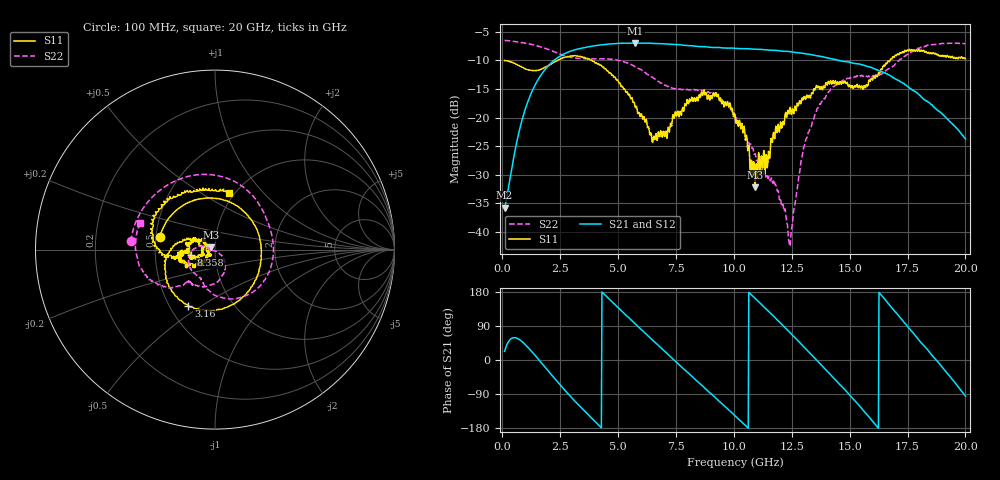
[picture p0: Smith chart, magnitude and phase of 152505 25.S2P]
!  2-Port S-parameters saved by WinCal
! VAR MeasName=S-Parameters (CALIBRATED_DATA) read from VNA (N5230C)
! VAR MeasDate=4/10/2015 9:30:51 AM
! VAR NAME=152505 25
! VAR FILENAME=152505 25.S2P
! VAR DATE=4/10/2015 9:30:51 AM
! VAR PHYS_PORTS=1,2
# Hz S DB R 50
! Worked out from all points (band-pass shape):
!   801 points, 100 MHz to 20 GHz, reference 50 ohm
!   highest |S21| = -6.97 dB at 5.747 GHz (marker M1); lowest = -35.7 dB at 100 MHz (marker M2)
!   |S21| within 3 dB of the highest: 2.252 GHz to 14.49 GHz (12.24 GHz wide, 146 % of centre)
!   lowest |S11| = -32.2 dB at 10.92 GHz (marker M3), VSWR 1.05, Z = 48 + j1.26 ohm
!   |S11| at or under -10 dB: start of sweep to 2.393 GHz; 3.863 GHz to 16.74 GHz (12.88 GHz wide, 125 % of centre)
!   |S22| runs from -42.5 to -6.5 dB; largest |S21 - S12| = 0.0073
!   S11 on the Smith chart (normalised r, x): 100 MHz: 0.53, +0.08; 3.16 GHz: 0.62, -0.44; 8.358 GHz: 0.76, -0.05; 20 GHz: 0.94, +0.67
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1e8  -10.05 166.8  -35.72 22.8  -35.60 22.2  -6.55 174.3
6.72125e8  -10.86 91.6  -23.40 56.3  -23.39 56.2  -6.80 142.2
1.44325e9  -11.79 5.7  -14.11 10.2  -14.11 10.2  -7.41 100.9
2.214375e9  -10.36 -55.5  -10.09 -45.4  -10.09 -45.4  -8.48 62.4
3.159625e9  -9.17 -115.3  -8.15 -110.2  -8.14 -110.3  -9.62 24.4
3.43325e9  -9.40 -130.4  -7.89 -127.5  -7.88 -127.5  -9.72 14.2
4.52775e9  -11.86 -176.8  -7.20 166.2  -7.21 166.0  -9.78 -28.9
5.746625e9  -18.29 156.5  -6.97 94.9  -7.03 94.9  -11.17 -78.3
6.741625e9  -22.49 -179.1  -7.08 38.2  -7.08 38.0  -13.73 -107.6
8.3585e9  -17.18 -167.8  -7.55 -52.9  -7.54 -52.5  -15.21 -135.3
9.179375e9  -16.28 166.8  -7.76 -98.0  -7.73 -98.0  -16.00 -159.6
1.005e10  -19.53 151.0  -7.91 -147.3  -7.93 -147.3  -19.82 172.8
1.092062e10  -32.20 147.5  -8.07 162.5  -8.07 162.8  -26.29 163.7
1.181612e10  -21.51 -131.8  -8.28 109.4  -8.28 108.9  -31.81 -167.5
1.2438e10  -18.22 -132.3  -8.52 71.3  -8.57 71.0  -42.37 -86.5
1.298525e10  -16.93 -139.2  -8.78 37.1  -8.81 37.0  -25.87 -42.9
1.338325e10  -15.76 -147.2  -9.06 12.1  -9.02 12.0  -20.83 -54.2
1.495038e10  -14.60 -174.7  -10.31 -88.9  -10.43 -89.0  -13.16 -109.9
1.589562e10  -13.69 -170.3  -11.18 -154.4  -11.15 -154.7  -12.78 -130.1
1.669162e10  -10.23 -176.9  -12.53 147.6  -12.59 146.5  -11.47 -131.7
1.823388e10  -8.52 130.6  -16.92 36.4  -16.89 36.0  -7.59 -162.9
2e10  -9.71 76.3  -23.72 -95.4  -23.73 -94.4  -7.09 160.7
